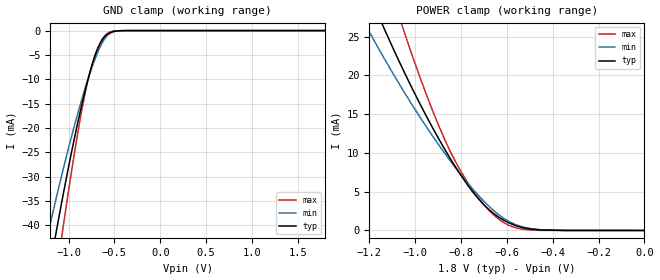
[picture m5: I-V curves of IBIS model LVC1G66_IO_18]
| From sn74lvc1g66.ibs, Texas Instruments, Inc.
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[Model]   LVC1G66_IO_18
Model_type  Terminator
| variable   typ   min   max
C_comp   10.09pF   4.65pF   28.59pF
| C_tri-state   10.09pF   4.65pF   28.59pF
[Temperature Range]   40   100   -40
| Ambient temperature   25   85   -40
[Voltage range]   1.8   1.65   1.95
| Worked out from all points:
|   GND clamp passes 1 mA (typ) near -0.59 V on its own axis
|   POWER clamp passes 1 mA (typ) near -0.59 V on its own axis
[GND Clamp]
| LVC1G66_IO_18
|   Voltage   I(typ)   I(min)   I(max)
-5.5V     -642.4mA   -532.1mA   -759.1mA
-1.225V   -50.88mA   -41.78mA   -62.75mA
-1.14V    -41.88mA   -34.83mA   -51.05mA
-1.08V    -35.76mA   -30.11mA   -43.06mA
-1.06V    -33.78mA   -28.57mA   -40.46mA
-910mV    -19.79mA   -17.72mA   -22.15mA
-795mV    -10.5mA    -10.36mA   -10.76mA
-685mV    -3.791mA   -4.563mA   -3.813mA
-585mV    -880.8uA   -1.18mA    -689.4uA
-505mV    -171uA     -215.7uA   -82.57uA
-375mV    -5.824uA   -8.939uA   -871.3nA
1.8V      88.84pA    48.31nA    18.88pA
[POWER Clamp]
| LVC1G66_IO_18
|   Voltage   I(typ)   I(min)   I(max)
-5.5V     592.3mA    476.9mA    790mA
-1.22V    31.87mA    26.7mA     42.11mA
-1.19V    29.77mA    25.08mA    39.05mA
-1.13V    25.69mA    21.93mA    33.16mA
-1.07V    21.82mA    18.92mA    27.58mA
-1.04V    19.95mA    17.47mA    24.91mA
-925mV    13.3mA     12.23mA    15.54mA
-825mV    8.235mA    8.129mA    8.922mA
-730mV    4.285mA    4.717mA    4.433mA
-640mV    1.81mA     2.137mA    1.566mA
-495mV    175uA      236.3uA    55.28uA
-95.1fV   88.84pA    700.1pA    22.15pA
